INTERFACE ICylinder

PROPERTY P_AtWorkPos : BOOL
SET
END_SET
GET
END_GET
END_PROPERTY

METHOD M_MoveToBase : BOOL
VAR_INPUT
END_VAR
END_METHOD

PROPERTY P_AtBasePos : BOOL
SET
END_SET
GET
END_GET
END_PROPERTY

METHOD M_Reset
VAR_INPUT
END_VAR
END_METHOD

METHOD M_StateMachine : BOOL
VAR_INPUT
	bBasePosReq		: BOOL;
	bWorkPosReq		: BOOL;
END_VAR
END_METHOD

PROPERTY P_ToWork : BOOL
SET
END_SET
GET
END_GET
END_PROPERTY

METHOD M_MoveToWork : BOOL
VAR_INPUT
END_VAR
END_METHOD

END_INTERFACE
